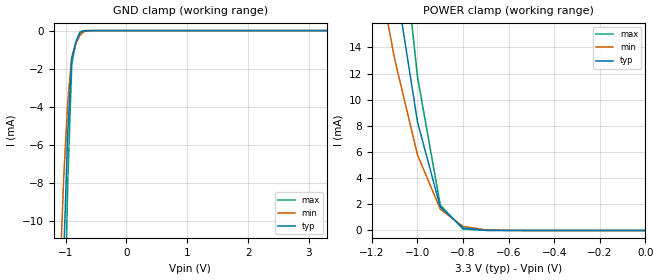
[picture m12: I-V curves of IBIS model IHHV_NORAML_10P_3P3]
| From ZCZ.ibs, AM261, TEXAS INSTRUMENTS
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[Model]   IHHV_NORAML_10P_3P3
Model_type   Input
Polarity   Non-Inverting
Vinl =  0.45
Vinh =  1.35
C_comp   0.8090088p   0.6964741p   0.9273633p
|[Input load] normal
|[supplytol] 10
|[temp] ind
[Model Spec]
Vinl   0.45   0.45   0.45
Vinh   1.35   1.35   1.35
[Temperature Range]   25   125   -40
[Voltage Range]   3.3   2.97   3.63
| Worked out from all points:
|   GND clamp passes 1 mA (typ) near -0.86 V on its own axis
|   POWER clamp passes 1 mA (typ) near -0.85 V on its own axis
| Nom Voltages:
|   VDD=1.1001, VDDS=3.3, VDDS18=1.8, BUS_VSSS=0, ESD_BIASFET=0, VSS=0
| Min Voltages:
|   VDD=0.99, VDDS=2.97, VDDS18=1.62, BUS_VSSS=0, ESD_BIASFET=0, VSS=0
| Max Voltages:
|   VDD=1.21, VDDS=3.63, VDDS18=1.98, BUS_VSSS=0, ESD_BIASFET=0, VSS=0
[POWER_clamp]
|   voltage   I(typ)   I(min)   I(max)
-3.3V     371.2mA    370.3mA    505mA
-1.133V   23.9mA     16.18mA    34.49mA
-1.1V     19.44mA    13.09mA    28.17mA
-1.067V   15.73mA    10.66mA    22.7mA
-1.033V   12.01mA    8.222mA    17.23mA
-1V       8.302mA    5.787mA    11.75mA
-900mV    1.797mA    1.632mA    1.94mA
-800mV    189uA      307.3uA    103.9uA
-700mV    15.91uA    49.24uA    4.319uA
-600mV    1.307uA    7.612uA    191.3nA
0V        882.7pA    1.774nA    3.92nA
[GND_clamp]
|   voltage   I(typ)   I(min)   I(max)
-3.3V     -581.8mA   -500.6mA   -861.2mA
-1.1V     -21.15mA   -13.37mA   -33.16mA
-1.033V   -11.94mA   -7.783mA   -18.55mA
-966.7mV  -5.39mA    -3.782mA   -8.085mA
-900mV    -1.486mA   -1.371mA   -1.752mA
-833.3mV  -616.2uA   -677.5uA   -645.7uA
-766.7mV  -124.3uA   -239.5uA   -62.58uA
-700mV    -10.21uA   -56.78uA   -2.085uA
-500mV    -38.4nA    -763.7nA   -6.11nA
3.3V      0A         0A         0A
